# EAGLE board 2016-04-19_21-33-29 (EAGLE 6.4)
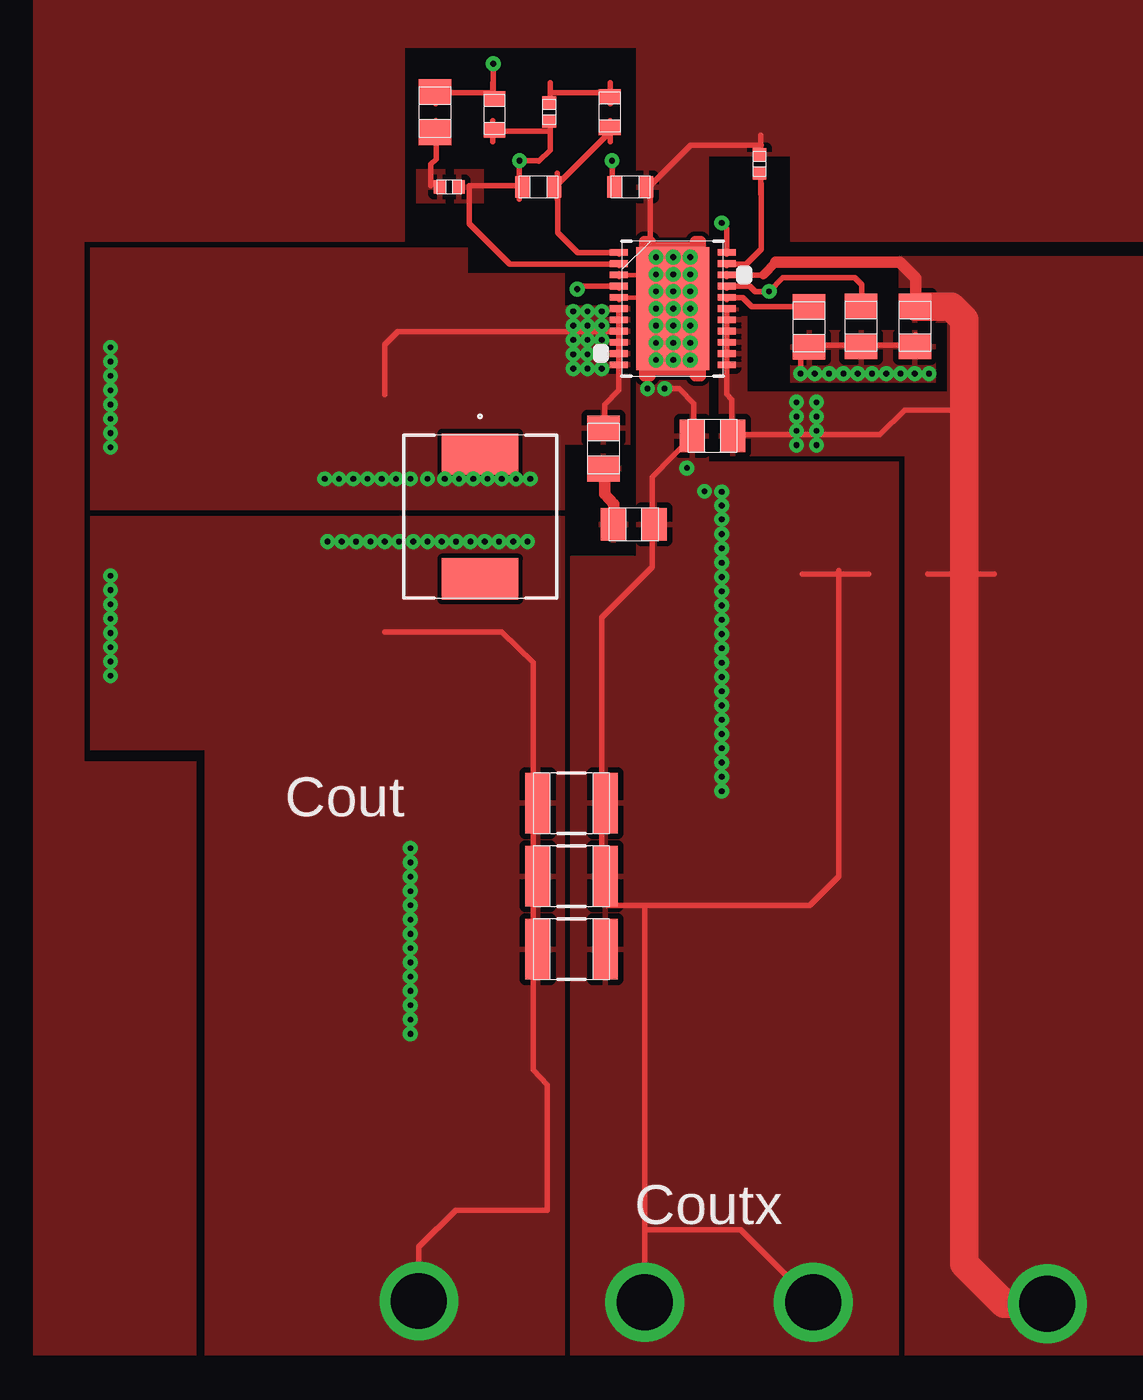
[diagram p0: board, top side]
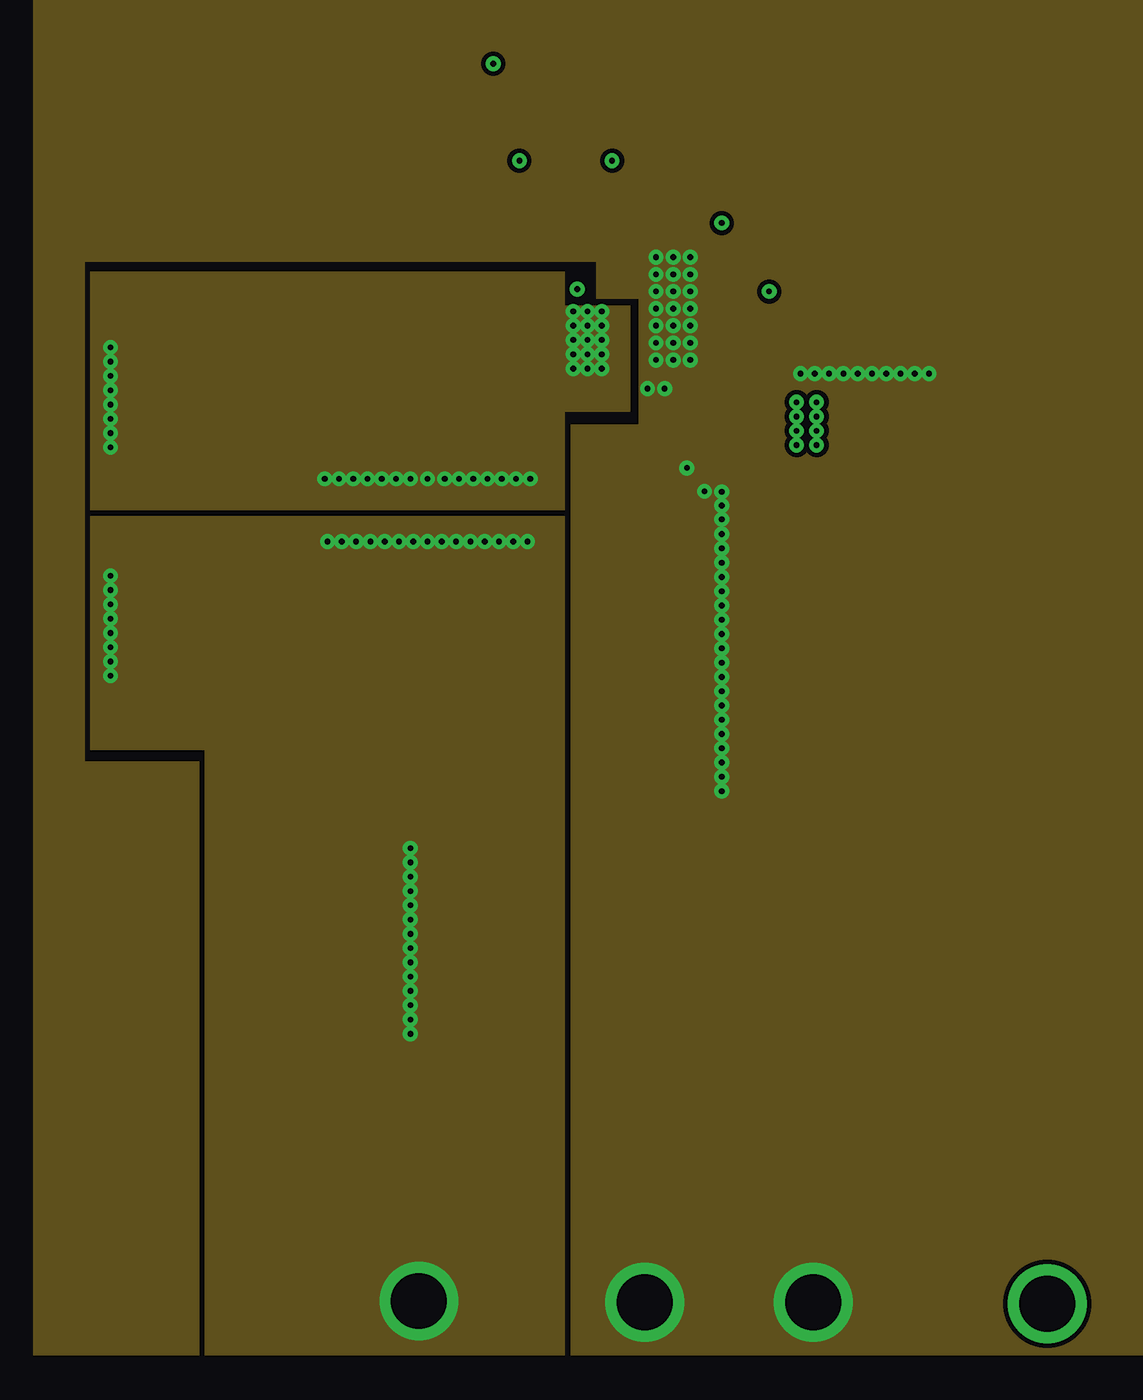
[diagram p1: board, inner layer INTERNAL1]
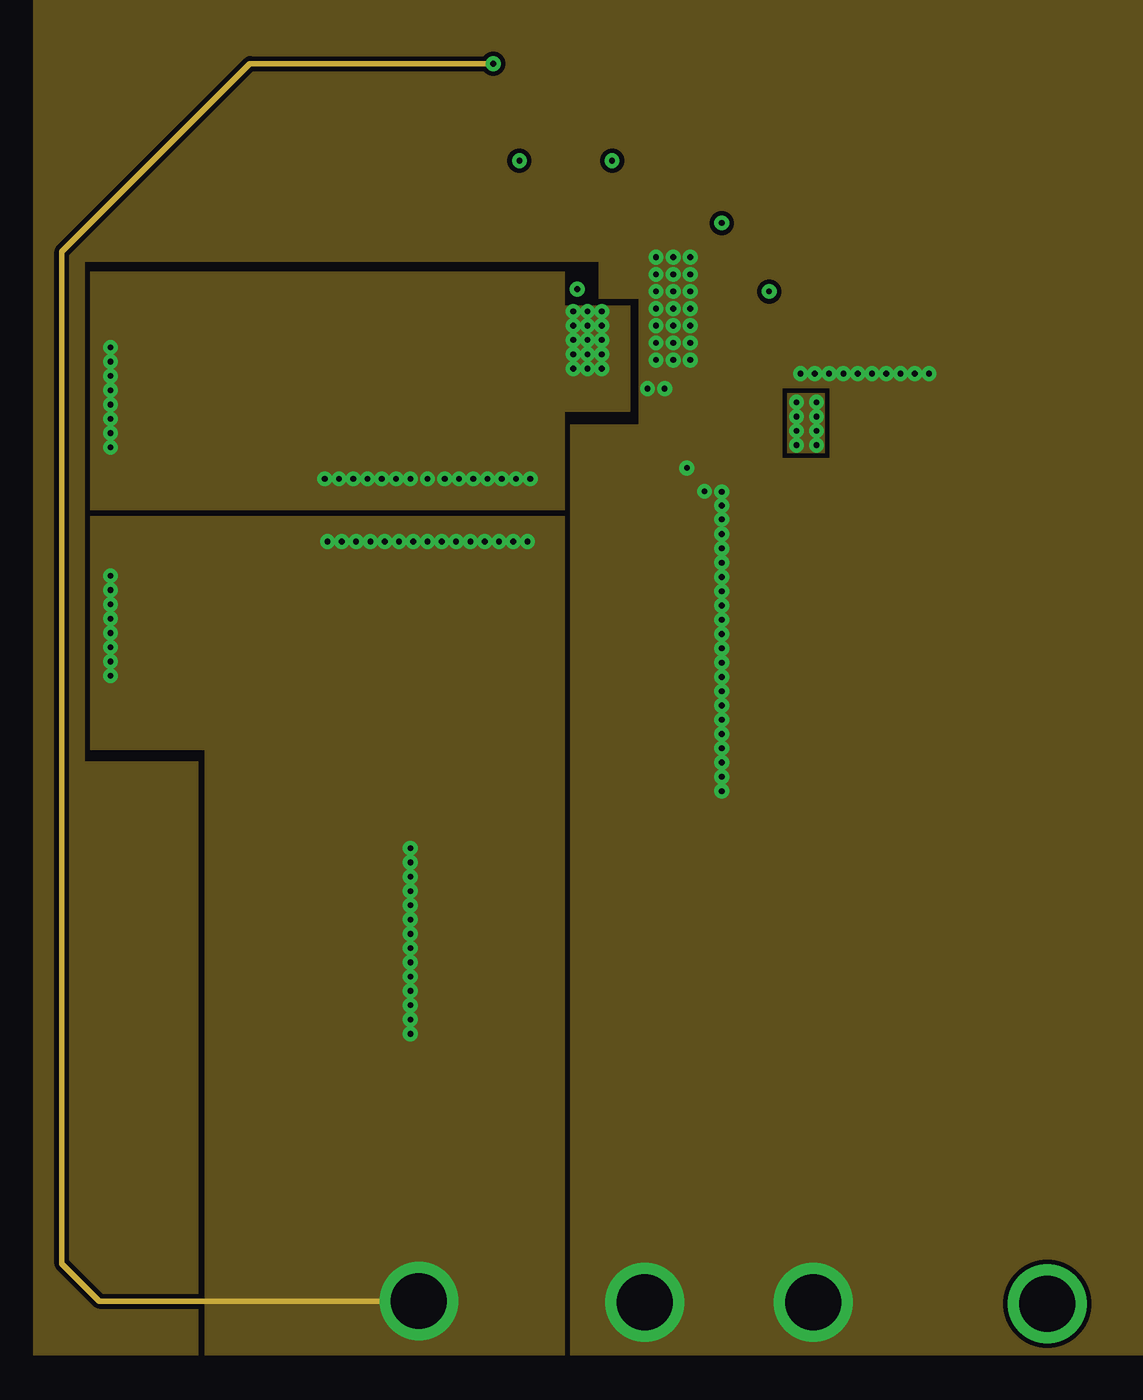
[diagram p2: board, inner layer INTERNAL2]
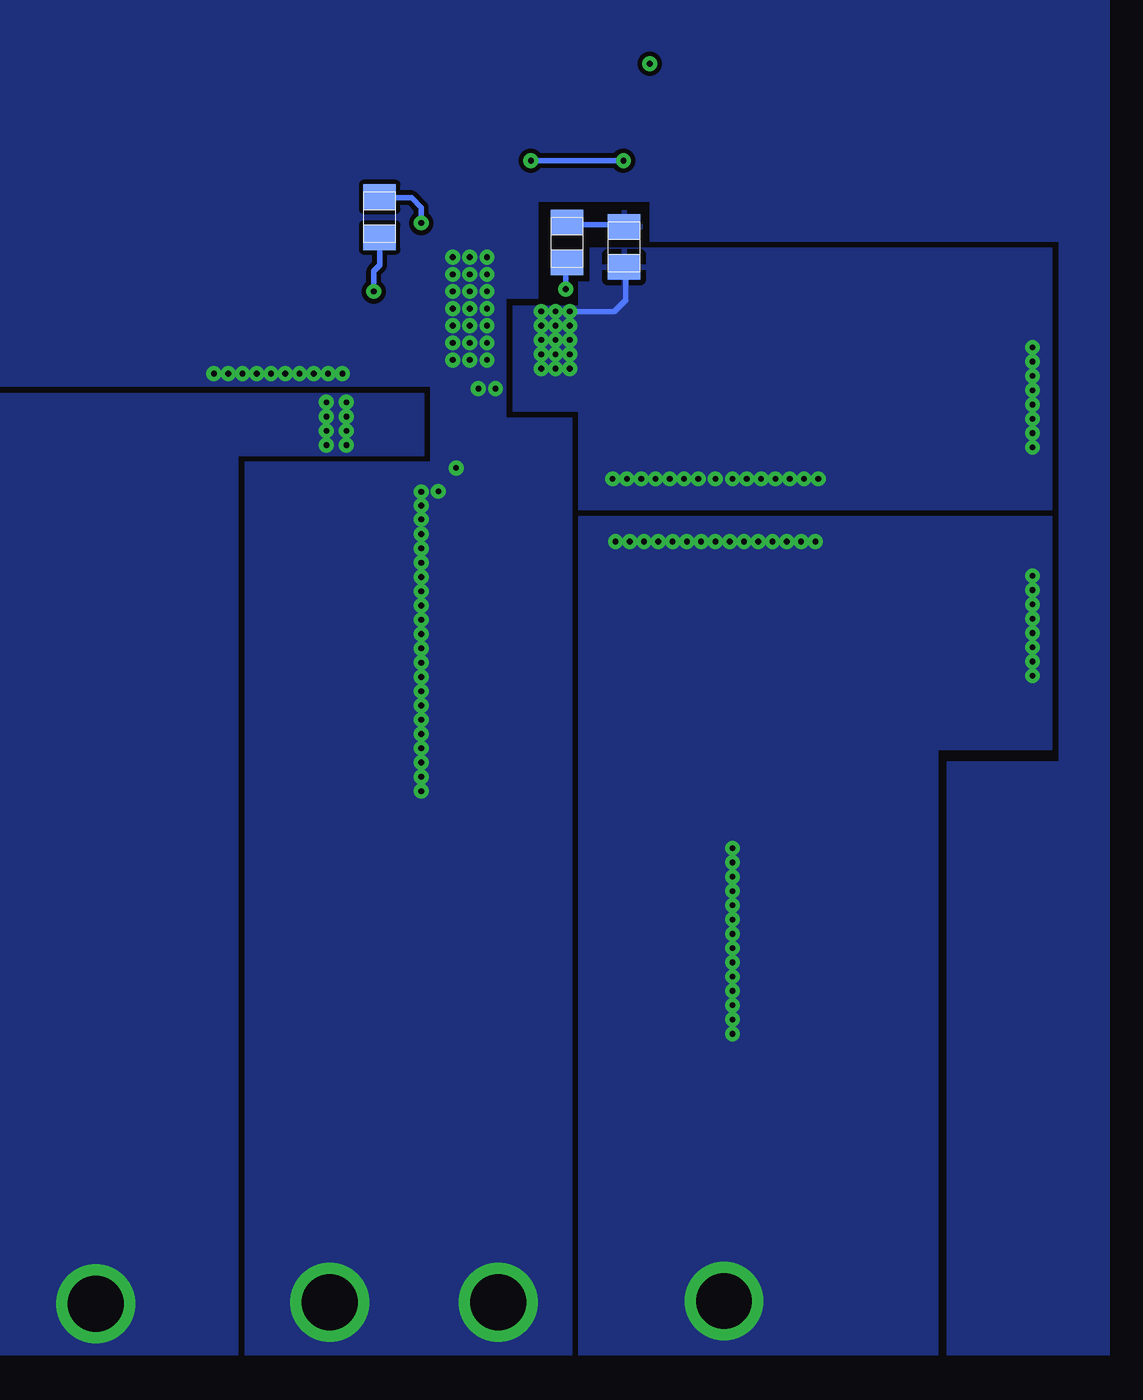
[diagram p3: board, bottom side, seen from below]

No outline drawn. Coordinates in mm, seen from the top.
Copper layers ((1*2)+(15*16)): TOP / INTERNAL1 / layer 15 / BOTTOM

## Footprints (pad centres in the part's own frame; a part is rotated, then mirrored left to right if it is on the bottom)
0805 = smd 1.118 x 1.448: 1 -0.902,0; 2 0.902,0
0603 = smd 0.66 x 0.965: 1 -0.699,0; 2 0.699,0
1210_280 = smd 1.118 x 2.692: 1 -1.499,0; 2 1.499,0
0402 = smd 0.559 x 0.61: 1 -0.419,0; 2 0.419,0
TP-1502 = drill 0.813 round: 1 0,0
CDEP63 = smd 1.841 x 3.404: 1 -2.775,0; 2 2.775,0
R-PSON-N22 = smd 0.805 x 0.305: 1 -2.402,2.5; 2 -2.402,2; 3 -2.402,1.5; 4 -2.402,1; 5 -2.402,0.5; 6 -2.402,0; 7 -2.402,-0.5; 8 -2.402,-1; 9 -2.402,-1.5; 10 -2.402,-2; 11 -2.402,-2.5; 12 2.402,-2.5; 13 2.402,-2; 14 2.402,-1.5; 15 2.402,-1; 16 2.402,-0.5; 17 2.402,0; 18 2.402,0.5; 19 2.402,1; 20 2.402,1.5; 21 2.402,2; 22 2.402,2.5 | smd 3.24 x 5.48: 23 0,0

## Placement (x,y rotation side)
Cboot  [0805]  47.62,75.34 90 bottom
Cbyp  [0805]  62.84,71.81 270 top
Ccomp  [0603]  51.66,81.33 270 top
CComp2  [0603]  48.49,78 180 top
Ccomp3  [0805]  43.89,81.33 270 top
Cin  [1206]  64.44,64.47 180 top
Cinx  [0805]  56.24,66.93 180 top
Cout_1  [1210_280]  49.96,50.6 0 top
Cout_2  [1210_280]  49.96,47.35 0 top
Cout_3  [1210_280]  49.96,44.09 0 top
Csnubber  [0805]  52.73,62.99 0 top
Css  [0402]  58.32,79.02 90 top
Cvcc  [0805]  65.23,71.81 270 top
GND  [TP-1502]  60.68,28.37 0 top
GND1  [TP-1502]  53.19,28.37 0 top
L1  [CDEP63]  45.9,63.35 270 top
Rcomp  [0402]  48.97,81.33 90 top
Rcomp2  [0402]  44.53,78 0 top
Rfbb  [0603]  52.58,78 0 top
Rfbt  [0603]  46.53,81.23 270 top
Rocset  [0805]  60.53,71.78 270 top
Rpgood  [0805]  58.5,76.66 90 bottom
Rramp  [0805]  50.16,75.54 270 bottom
Rsnubber  [0805]  51.38,66.37 90 top
U1  [R-PSON-N22]  54.46,72.59 0 top
VIN  [TP-1502]  71.09,28.3 0 top
VOUT  [TP-1502]  43.13,28.45 0 top

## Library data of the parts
Cboot = ultra-librarian; RefDes: Cboot; Type: C0805C104K5RACTU
Cbyp = ultra-librarian; RefDes: Cbyp; Type: GRM21BR61E475KA12L
Ccomp = ultra-librarian; RefDes: Ccomp; Type: C0603C682K5RACTU
CComp2 = ultra-librarian; RefDes: CComp2; Type: CL10C122JB8NNNC
Ccomp3 = ultra-librarian; RefDes: Ccomp3; Type: CL21C102JBCNFNC
Cin = ultra-librarian; RefDes: Cin; Type: C3216X5R1E476M160AC
Cinx = ultra-librarian; RefDes: Cinx; Type: GRM219R71E105KA88D
Cout_1-Cout_3 = ultra-librarian
Csnubber = ultra-librarian; RefDes: Csnubber; Type: C0805C222K5RACTU
Css = ultra-librarian; RefDes: Css; Type: GRM155R71C153KA01D
Cvcc = ultra-librarian; RefDes: Cvcc; Type: GRM219R71E105KA88D
GND = ultra-librarian; RefDes: GND; Type: TP-1502
GND1 = ultra-librarian; RefDes: GND1; Type: TP-1502
L1 = ultra-librarian; RefDes: L1; Type: CDEP63MENP-R68MC
Rcomp = ultra-librarian; RefDes: Rcomp; Type: CRCW04023K24FKED
Rcomp2 = ultra-librarian; RefDes: Rcomp2; Type: CRCW04023K57FKED
Rfbb = ultra-librarian; RefDes: Rfbb; Type: RC0603FR-0733KL
Rfbt = ultra-librarian; RefDes: Rfbt; Type: RC0603FR-0722KL
Rocset = ultra-librarian; RefDes: Rocset; Type: ERJ-6ENF1781V
Rpgood = ultra-librarian; RefDes: Rpgood; Type: ERJ-6ENF1003V
Rramp = ultra-librarian; RefDes: Rramp; Type: CRCW08055R11FKEA
Rsnubber = ultra-librarian; RefDes: Rsnubber; Type: CRCW08051R00FKEA
U1 = ultra-librarian; RefDes: U1; Type: TPS56121DQPR
VIN = ultra-librarian; RefDes: VIN; Type: TP-1502
VOUT = ultra-librarian; RefDes: VOUT; Type: TP-1502

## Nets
0: Cbyp.2 Cin.2 Cinx.2 Cout_1.2 Cout_2.2 Cout_3.2 Csnubber.2 Css.2 Cvcc.2 GND1.1 GND.1 Rfbb.2 Rocset.2 U1.3 U1.5 U1.23
1: Cin.1 Cinx.1 Cvcc.1 U1.12 U1.13 U1.14 U1.15 U1.16 U1.17 U1.20 VIN.1
2: Cbyp.1 Rpgood.1 U1.19
4: CComp2.1 Ccomp.2 U1.1
5: Cboot.1 L1.2 Rsnubber.2 U1.6 U1.7 U1.8 U1.9 U1.10 U1.11
6: CComp2.2 Rcomp2.2 Rcomp.1 Rfbb.1 Rfbt.2 U1.2
8: Ccomp3.1 Cout_1.1 Cout_2.1 Cout_3.1 L1.1 Rfbt.1 VOUT.1
10: Rramp.2 U1.4
11: Ccomp.1 Rcomp.2
12: Ccomp3.2 Rcomp2.1
13: Cboot.2 Rramp.1
14: Csnubber.1 Rsnubber.1
20: Rpgood.2 U1.22
21: Css.1 U1.21
28: Rocset.1 U1.18

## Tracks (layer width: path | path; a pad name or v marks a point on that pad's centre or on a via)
0  (via drill 0.25 pad 0.56, 2.49 pad 3.48)
  TOP 0.203: 52.07,73.08 52.98,73.08 53.49,72.59 v53.72,72.59 v54.48,72.59 v53.72,73.36 52.98,74.09 U1.3
  TOP 0.254: v53.21,28.4 53.21,46.05 | 53.34,31.62 57.48,31.62 v60.71,28.4 | 53.21,46.05 60.55,46.05 61.85,47.35 61.85,60.94 | 53.21,46.05 51.56,46.05 51.31,46.3 51.31,55.19 51.31,58.85 53.54,61.09 53.54,62.94 53.54,65.1 55.4,66.98 55.4,68.38 54.76,69.04 v54.1,69.04 | 58.4,79.86 55.27,79.86 53.47,78.05 53.47,74.57 52.98,74.09 | 65.28,70.97 | v60.15,69.7 60.15,70.66 60.45,70.97 65.28,70.97 | 65.27,70.48 65.27,71.42 | 62.28,70.95 63.42,70.95 | 58.38,79.38 58.38,80.31 | 55.38,66.4 55.38,67.54 | 51.31,48.9 51.31,51.33 | 60.22,60.78 63.17,60.78 | 54.47,69.75 54.47,75.39 | 52.08,73.13 52.08,73 | 52.08,74.14 52.08,74.02
  other vias: 55.88,64.47 55.09,65.51 56.64,56.21 56.64,63.83 55.24,72.59 65.23,69.7 56.64,51.13 56.64,54.31 56.64,53.67 56.64,53.04 56.64,52.4 56.64,51.77 56.64,54.94 56.64,55.58 56.64,56.85 56.64,58.12 56.64,58.75 56.64,59.39 56.64,60.02 56.64,60.66 56.64,61.29 56.64,61.93 56.64,62.56 56.64,63.22 56.64,57.48 65.86,69.7 64.59,69.7 63.96,69.7 62.05,69.7 61.42,69.7 60.78,69.7 62.69,69.7 63.32,69.7 56.64,64.44 53.72,70.31 53.72,71.07 53.72,71.83 54.48,70.31 54.48,71.07 54.48,71.83 53.34,69.04 55.24,73.36 55.24,74.12 55.24,74.88 53.72,74.12 54.48,74.88 54.48,74.12 54.48,73.36 55.24,71.83 53.72,74.88 55.24,71.07 55.24,70.31
  pour TOP (rank 5): 59.69,71.63 59.69,69.29 66.17,69.29 66.17,71.63
  pour TOP (rank 6): 52.88,72.69 52.88,69.62 56.08,69.62 56.08,72.69
  pour TOP (rank 6): 49.91,26.04 49.91,61.59 52.83,61.59 52.83,84.2 42.55,84.2 42.55,75.56 28.3,75.56 28.3,52.45 33.27,52.45 33.27,26.04 26.04,26.04 26.04,97.79 88.27,97.79 88.27,26.04 75.95,26.04 75.95,75.56 59.69,75.56 59.69,79.38 56.06,79.38 56.06,65.79 64.52,65.79 64.52,26.04
  pour BOTTOM (rank 5): 26.04,97.79 88.27,97.79 88.27,26.04 75.97,26.04 75.97,69.11 56.24,69.11 56.24,65.79 64.49,65.79 64.49,26.04 49.94,26.04 49.94,67.74 52.86,67.74 52.86,73.03 51.44,73.03 51.44,77.34 46.48,77.34 46.48,75.56 28.3,75.56 28.3,52.45 33.27,52.45 33.27,26.04 26.04,26.04
  pour INTERNAL1 (rank 5): 26.04,97.79 88.27,97.79 88.27,26.04 49.94,26.04 49.94,67.44 52.96,67.44 52.96,73.03 51.05,73.03 51.05,74.68 28.32,74.68 28.32,52.45 33.4,52.45 33.4,26.04 26.04,26.04
  pour INTERNAL2 (rank 5): 26.04,97.74 88.27,97.74 88.27,26.04 49.91,26.04 49.91,67.44 52.96,67.44 52.96,73.03 51.18,73.03 51.18,74.68 28.32,74.68 28.32,52.45 33.38,52.45 33.38,26.04 26.04,26.04
1  (via drill 0.25 pad 0.56, 2.49 pad 3.48)
  TOP 0.254: 67.44,68.07 64.77,68.07 63.68,66.98 57.1,66.98 57.1,68.56 56.87,68.78 56.87,70.08 56.87,70.59 56.87,71.07 56.87,71.58 56.87,72.08 56.87,72.59 | 56.87,74.09 58.5,74.09 | 65.27,72.19 65.27,73.13 | 57.09,66.4 57.09,67.54 | 65.81,60.78 68.76,60.78 | 56.86,72.64 56.86,72.52 | 56.86,70.13 56.86,70 | 56.86,72.14 56.86,72.01 | 56.86,71.63 56.86,71.5 | 56.86,71.14 56.86,71.02 | 56.86,70.64 56.86,70.51 | 56.86,74.14 56.86,74.02
  TOP 0.381: 58.5,74.09 59.05,74.65
  TOP 0.508: 65.28,72.67 65.28,73.94 64.57,74.65 59.05,74.65
  TOP 1.27: v71.12,28.32 69.22,28.32 67.44,30.1 67.44,68.07 67.44,72.11 66.85,72.67 65.28,72.67
  other vias: 60.86,67.16 60.86,66.52 60.86,67.79 59.97,68.43 59.97,67.79 59.97,67.16 59.97,66.52 60.86,68.43
  pour TOP (rank 4): 64.77,26.04 64.77,66.04 56.52,66.04 56.52,72.64 57.4,72.64 57.4,72.26 57.78,72.26 57.78,68.91 66.67,68.91 66.67,71.96 64.52,71.96 64.52,74.93 75.69,74.93 75.69,26.04
  pour BOTTOM (rank 2): 64.77,26.04 64.77,66.04 56.52,66.04 56.52,68.83 75.69,68.83 75.69,26.04
  pour INTERNAL2 (rank 3): 59.56,68.83 61.21,68.83 61.21,66.17 59.56,66.17
2  (via drill 0.25 pad 0.56)
  TOP 0.254: 56.87,73.58 57.89,73.58 58.14,73.36 v58.75,73.36 59.36,73.97 62.56,73.97 62.87,73.66 62.87,72.67 | 62.28,72.66 63.42,72.66 | 56.86,73.64 56.86,73.51
  BOTTOM 0.254: 58.5,75.82 58.5,74.52 58.75,74.27 v58.75,73.36 | 57.91,75.81 59.05,75.81
4
  TOP 0.254: 51.69,80.47 49.35,78.13 49.35,78.05 49.35,75.97 50.24,75.08 U1.1 | 51.68,80.01 51.68,80.95 | 49.34,77.47 49.34,78.61 | 52.08,75.13 52.08,75.01
5  (via drill 0.25 pad 0.56)
  TOP 0.254: 52.07,71.58 42.24,71.58 41.66,70.99 41.66,68.76 | 51.44,67.21 51.44,68.33 52.07,68.96 52.07,70.08 U1.10 52.07,71.07 52.07,71.58 | 52.07,71.58 U1.7 U1.6 | 52.08,72.64 52.08,72.52 | 52.08,70.13 52.08,70 | 52.08,70.64 52.08,70.51 | 52.08,71.14 52.08,71.02 | 52.08,71.63 52.08,71.5 | 52.08,72.14 52.08,72.01
  BOTTOM 0.254: 47.55,74.62 47.55,72.97 48.06,72.47 49.02,72.47 v50.04,72.47
  other vias: 29.46,68.96 29.46,68.33 29.46,70.87 29.46,69.6 29.46,67.06 29.46,66.42 29.46,67.69 29.46,70.23 44.32,65.02 44.96,65.02 45.59,65.02 46.23,65.02 46.86,65.02 47.5,65.02 48.13,65.02 43.56,65.02 51.31,71.83 50.67,71.83 50.67,72.47 51.31,72.47 50.67,70.56 50.67,71.2 50.67,69.93 50.04,69.93 51.31,69.93 51.31,70.56 51.31,71.2 50.04,70.56 50.04,71.83 50.04,71.2 42.8,65.02 42.16,65.02 41.53,65.02 40.89,65.02 40.26,65.02 39.62,65.02 38.99,65.02
  pour TOP (rank 4): 28.57,75.31 28.57,63.63 49.66,63.63 49.66,66.55 52.58,66.55 52.58,72.72 49.66,72.72 49.66,74.17 45.34,74.17 45.34,75.31
  pour BOTTOM (rank 3): 28.57,63.63 49.66,63.63 49.66,68.02 52.58,68.02 52.58,72.72 49.66,72.72 49.66,73.79 49.15,73.79 49.15,75.31 28.57,75.31
  pour INTERNAL1 (rank 2): 28.57,74.24 28.57,63.63 49.66,63.63 49.66,68.02 52.58,68.02 52.58,72.72 49.66,72.72 49.66,74.24
  pour INTERNAL2 (rank 4): 28.57,74.24 28.57,63.63 49.66,63.63 49.66,68.02 52.58,68.02 52.58,72.72 49.66,72.72 49.66,74.24
6  (via drill 0.25 pad 0.56)
  TOP 0.254: 48.51,79.15 49.02,79.63 49.02,80.49 46.48,80.49 | v47.65,79.17 48.51,79.17 | 47.65,79.15 47.65,78.05 45.41,78.05 45.41,76.38 47.22,74.57 52.07,74.57 | 51.77,78.05 v51.77,79.17 | 46.47,80.01 46.47,80.95 | 49.01,80.01 49.01,80.95 | 47.64,77.47 47.64,78.61 | 52.08,74.62 52.08,74.5
  BOTTOM 0.254: v47.65,79.17 v51.77,79.17 | v47.65,79.17
  pour TOP: 44.75,77.29 44.75,78.79 46.05,78.79 46.05,77.29
8  (via drill 0.25 pad 0.56, 2.49 pad 3.48)
  TOP 0.254: v43.18,28.45 43.18,30.86 44.81,32.49 48.9,32.49 48.9,38.08 48.26,38.73 48.26,50.11 48.26,56.84 46.86,58.22 41.66,58.22 | v46.48,83.49 46.48,82.19 43.94,82.19 | 43.93,81.71 43.93,82.65 | 46.47,81.71 46.47,82.65 | 48.26,48.9 48.26,51.33
  INTERNAL2 0.254: v43.18,28.45 28.96,28.45 27.3,30.1 27.3,75.13 35.66,83.49 v46.48,83.49
  other vias: 41.66,62.23 43.56,62.23 42.29,62.23 40.39,62.23 39.75,62.23 39.12,62.23 48.01,62.23 42.8,46.05 42.8,45.42 42.8,44.78 42.8,44.15 42.8,43.51 42.8,42.88 42.8,42.24 42.8,41.61 42.8,40.97 42.8,40.34 42.8,48.59 42.8,47.96 42.8,47.32 42.8,46.69 47.37,62.23 46.74,62.23 46.1,62.23 45.47,62.23 44.83,62.23 44.2,62.23 29.46,60.07 29.46,57.53 29.46,56.26 29.46,56.9 29.46,59.44 29.46,60.71 29.46,58.17 41.02,62.23 42.93,62.23 29.46,58.8
  pour TOP (rank 4): 33.66,26.04 49.66,26.04 49.66,63.37 28.57,63.37 28.57,52.96 33.66,52.96
  pour BOTTOM (rank 3): 33.66,26.04 49.66,26.04 49.66,63.37 28.57,63.37 28.57,52.96 33.66,52.96
  pour INTERNAL1 (rank 2): 33.66,26.04 49.66,26.04 49.66,63.37 28.57,63.37 28.57,52.96 33.66,52.96
  pour INTERNAL2 (rank 3): 33.66,26.04 49.66,26.04 49.66,63.37 28.57,63.37 28.57,52.96 33.66,52.96
10  (via drill 0.25 pad 0.56)
  TOP 0.254: v50.22,73.46 50.34,73.58 U1.4 | 52.08,73.64 52.08,73.51
  BOTTOM 0.254: 50.22,74.65 v50.22,73.46 50.22,73.61
11
  TOP 0.254: 49.02,82.19 51.69,82.19 | 49.01,81.71 49.01,82.65 | 51.68,81.71 51.68,82.65
12
  TOP 0.254: 43.71,78.05 43.71,79.02 43.94,79.25 43.94,80.49 | 43.93,80.01 43.93,80.95
  pour TOP: 43.05,77.29 43.05,78.79 44.35,78.79 44.35,77.29
13
  BOTTOM 0.254: 47.55,76.33 50.14,76.33
  pour BOTTOM: 46.79,75.67 46.79,76.96 48.29,76.96 48.29,75.67
14
  TOP 0.508: 51.44,65.51 51.44,64.34 51.84,63.91 51.84,62.94
  pour TOP: 51.18,62.18 51.18,63.68 52.48,63.68 52.48,62.18
  pour TOP (rank 2): 50.67,64.85 50.67,66.14 52.17,66.14 52.17,64.85
20  (via drill 0.25 pad 0.56)
  TOP 0.254: v56.64,76.4 56.87,76.15 56.87,75.08 | 56.86,75.13 56.86,75.01
  BOTTOM 0.254: 58.5,77.52 57.07,77.52 56.64,77.09 v56.64,76.4 | 57.91,77.51 59.05,77.51
21
  TOP 0.254: 56.87,74.57 57.73,74.57 58.4,75.23 58.4,78.16 | 58.38,77.67 58.38,78.61 | 56.86,74.62 56.86,74.5
28
  TOP 0.254: 60.45,72.67 57.99,72.67 57.58,73.08 56.87,73.08 | 56.86,73.13 56.86,73

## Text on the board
ASSYNOTES: Cout | Coutx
